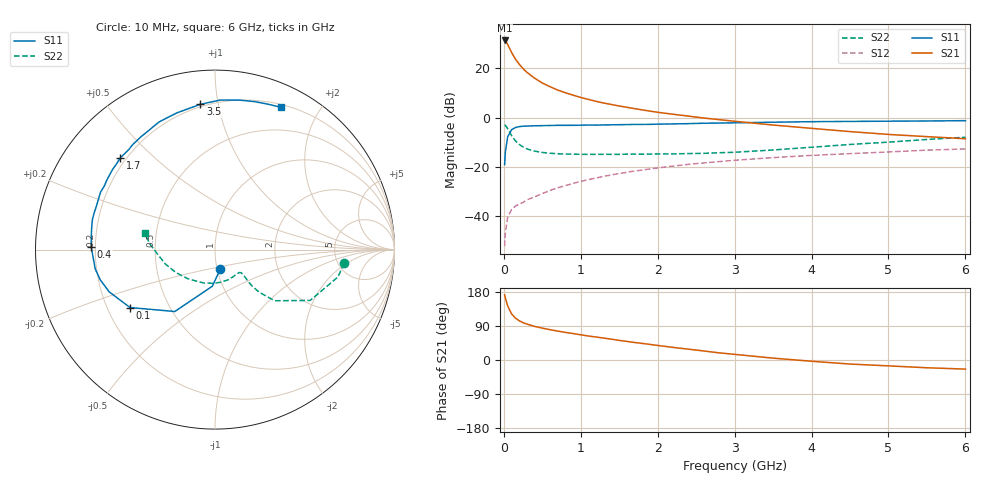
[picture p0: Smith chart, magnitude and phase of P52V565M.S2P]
! SIEMENS Small Signal Semiconductors
! BFP183
! Si NPN RF Bipolar Junction Transistor in SOT143
! VCE = 2.5 V  IC = 65 mA
! Common Emitter S-Parameters:  March  1996
# GHz  S  MA  R  50
!  f  S11  S21  S12  S22
! GHz  MAG  ANG  MAG  ANG  MAG  ANG  MAG  ANG
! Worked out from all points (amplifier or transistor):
!   36 points, 10 MHz to 6 GHz, reference 50 ohm
!   highest |S21| = 31.3 dB at 10 MHz (marker M1)
!   |S21| within 3 dB of that: start of sweep to 71.19 MHz
!   unconditionally stable (mu >= 1): start of sweep to 35.05 MHz; 164.7 MHz to end of sweep
!   at 250 MHz: K = 1.25, MAG = 24.1 dB, |S12| = -34.3 dB
!   at 1.4 GHz: K = 1.75, MAG = 9.2 dB, |S12| = -23.1 dB
!   at 6 GHz: K = 1.34, MAG = -1.4 dB, |S12| = -12.6 dB
!   S11 on the Smith chart (normalised r, x): 10 MHz: 1.04, -0.23; 100 MHz: 0.30, -0.28; 400 MHz: 0.18, +0.01; 1.7 GHz: 0.18, +0.39; 3.5 GHz: 0.19, +0.89; 6 GHz: 0.23, +1.54
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0.01  0.1125 -74.7  36.93 171.7  0.0025 61.1  0.7226 -6.0
0.02  0.2047 -94.2  36.16 163.5  0.0047 67.6  0.7023 -12.5
0.05  0.4113 -123.0  30.53 142.7  0.0097 62.2  0.6012 -28.1
0.1  0.5729 -145.7  21.18 121.9  0.0138 47.1  0.438 -40.6
0.15  0.6346 -158.2  15.57 110.6  0.0162 46.8  0.3425 -44.0
0.2  0.6614 -165.3  12.18 103.5  0.0178 47.8  0.2886 -44.5
0.25  0.676 -170.9  9.904 98.4  0.0193 49.5  0.2565 -43.8
0.3  0.6789 -175.2  8.344 94.8  0.0217 51.8  0.2342 -42.8
0.4  0.6894 178.9  6.352 88.7  0.025 54.7  0.2108 -41.7
0.5  0.693 174.2  5.078 84.1  0.0291 56.7  0.1983 -41.5
0.6  0.6981 169.7  4.272 80.0  0.0337 59.2  0.1913 -42.1
0.7  0.7033 166.1  3.649 76.3  0.0381 60.9  0.1867 -43.3
0.9  0.704 159.5  2.875 69.8  0.0468 62.0  0.1832 -47.1
1.1  0.7135 153.2  2.358 63.3  0.056 61.6  0.1814 -51.6
1.3  0.7163 147.4  1.987 57.7  0.065 61.1  0.182 -57.1
1.7  0.7342 136.1  1.532 46.2  0.0835 58.4  0.1833 -69.1
2.2  0.7517 123.3  1.18 33.2  0.1052 53.8  0.1851 -85.9
2.8  0.7825 109.4  0.916 18.8  0.1294 47.3  0.1959 -107.9
3.5  0.8134 95.8  0.713 4.9  0.1559 40.1  0.2227 -133.5
4.5  0.8441 80.6  0.525 -10.7  0.1878 29.4  0.288 -163.8
5.5  0.8618 70.2  0.415 -20.5  0.2209 20.0  0.3638 175.2
6  0.8738 65.2  0.376 -24.0  0.2338 14.7  0.4029 166.7
